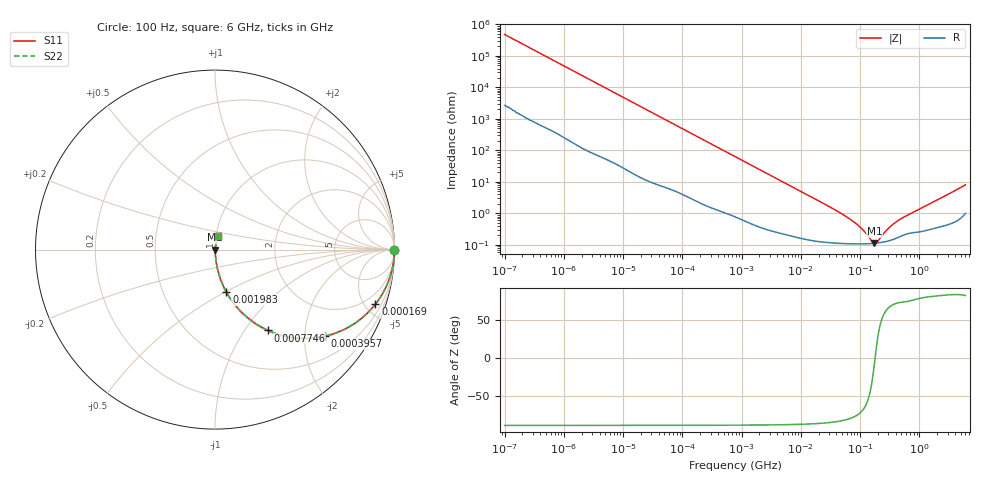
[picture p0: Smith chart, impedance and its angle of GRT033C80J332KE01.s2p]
!Murata Part Number: GRT033C80J332KE01
!These Parameters are Measured in Series Mode Connection
!Data Generated on Jun 19, 2026
!  o--ll--o
!Port1  Port2
!  o------o
!Operation Temp=25[degC], DC Bias Voltage=0[V]
!Freq. Start=100[Hz] Stop=6[GHz] 401[Steps]
# Hz S RI R 50
!Freq.(Hz) S11(Real) S11(Imag) S21(Real) S21(Imag) S12(Real) S12(Imag) S22(Real) S22(Imag)
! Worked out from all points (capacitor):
!   401 points, 100 Hz to 6 GHz, reference 50 ohm
!   read as one part in series: C = 3.3 nF near 109 Hz
!   lowest |Z| = 114 mohm at 174.6 MHz (marker M1)
!   series resonance near 179.5 MHz, so ESL is about 240 pH
!   S11 on the Smith chart (normalised r, x): 100 Hz: open; 169 kHz: 1.05, -5.85; 395.7 kHz: 1.03, -2.51; 774.6 kHz: 1.02, -1.29; 1.983 MHz: 1.01, -0.51; 6 GHz: 1.02, +0.16
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100  1 -0.000208  1.2e-06 0.000208  1.2e-06 0.000208  1 -0.000208
2008  1 -0.00413  3.74e-05 0.00413  3.74e-05 0.00413  1 -0.00413
12592  0.9992 -0.0257  0.000806 0.0257  0.000806 0.0257  0.9992 -0.0257
40335  0.9928 -0.0815  0.00722 0.0815  0.00722 0.0815  0.9928 -0.0815
86348  0.9689 -0.1695  0.0311 0.1695  0.0311 0.1695  0.9689 -0.1695
169018  0.8934 -0.3044  0.1066 0.3044  0.1066 0.3044  0.8934 -0.3044
252896  0.7912 -0.402  0.2088 0.402  0.2088 0.402  0.7912 -0.402
395726  0.6105 -0.4826  0.3895 0.4826  0.3895 0.4826  0.6105 -0.4826
774597  0.2955 -0.4502  0.7045 0.4502  0.7045 0.4502  0.2955 -0.4502
1212075  0.149 -0.3496  0.851 0.3496  0.851 0.3496  0.149 -0.3496
1983483  0.0633 -0.2363  0.9367 0.2363  0.9367 0.2363  0.0633 -0.2363
4856642  0.0129 -0.1024  0.9871 0.1024  0.9871 0.1024  0.0129 -0.1024
1.555665e7  0.00242 -0.0324  0.9976 0.0324  0.9976 0.0324  0.00242 -0.0324
4.165952e7  0.00127 -0.0116  0.9987 0.0116  0.9987 0.0116  0.00127 -0.0116
7.455971e7  0.00111 -0.0057  0.9989 0.0057  0.9989 0.0057  0.00111 -0.0057
1.066761e8  0.00109 -0.00312  0.9989 0.00312  0.9989 0.00312  0.00109 -0.00312
1.596157e8  0.00111 -0.000672  0.9989 0.000672  0.9989 0.000672  0.00111 -0.000672
1.745687e8  0.00113 -0.000157  0.9989 0.000157  0.9989 0.000157  0.00113 -0.000157
1.996653e8  0.00116 0.000613  0.9988 -0.000613  0.9988 -0.000613  0.00116 0.000613
3.124326e8  0.00137 0.00331  0.9986 -0.00331  0.9986 -0.00331  0.00137 0.00331
5.59173e8  0.00215 0.0075  0.9979 -0.0075  0.9979 -0.0075  0.00215 0.0075
6e9  0.0162 0.0783  0.9838 -0.0783  0.9838 -0.0783  0.0162 0.0783
